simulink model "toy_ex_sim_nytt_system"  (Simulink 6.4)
settings: Solver=ode4  StartTime=0.0  StopTime=200  RelTol=1e-5
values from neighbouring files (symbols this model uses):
  alpha = -0.9    [bounds.m]    (also in real_ex_linkomb_W_and_DP.m = 1; real_ex_linkomb_W_and_RHOT.m = -0.2; real_ex_without_noise_z_30.m = -6:0.01:4; toy_ex_nytt_system.m)
  den_G1 = [-1 1]    [bounds.m]    (also in toy_ex_nytt_system.m; toy_ex_nytt_system_without_noise.m; toy_ex_nytt_system_with_disturbance.m; toy_ex_nytt_system_with_measure_noise.m)
  den_G2 = [-1 1]    [bounds.m]    (also in toy_ex_nytt_system.m; toy_ex_nytt_system_without_noise.m; toy_ex_nytt_system_with_disturbance.m; toy_ex_nytt_system_with_measure_noise.m)
  K = 2    [toy_ex_OLD.m]
  K_indre = 10    [real_ex_linkomb_W_and_DP.m]    (also in real_ex_linkomb_W_and_RHOT.m = 5; toy_ex_nytt_system.m = 50; toy_ex_nytt_system_without_noise.m = 20; toy_ex_nytt_system_with_disturbance.m = 50)
  num_G1 = 5*[-1.5 1]    [bounds.m]    (also in toy_ex_nytt_system.m; toy_ex_nytt_system_without_noise.m; toy_ex_nytt_system_with_disturbance.m; toy_ex_nytt_system_with_measure_noise.m)
  num_G2 = 5*[-0.5 1]    [bounds.m]    (also in toy_ex_nytt_system.m; toy_ex_nytt_system_without_noise.m; toy_ex_nytt_system_with_disturbance.m; toy_ex_nytt_system_with_measure_noise.m)
undefined symbols (not defined in the file or in its folder): Ti_indre

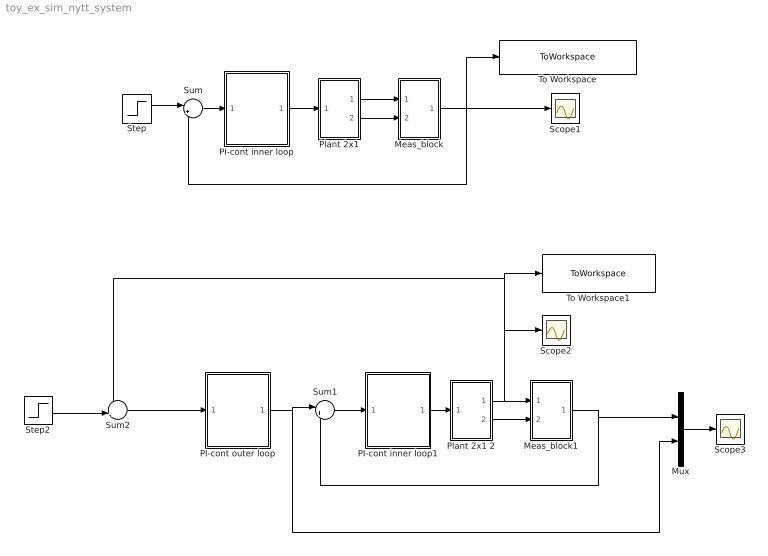
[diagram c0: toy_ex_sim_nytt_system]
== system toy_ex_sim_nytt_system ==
  Meas_block : Subsystem
  Meas_block1 : Subsystem
  Mux : Mux  Inputs=2
  PI-cont inner loop : Subsystem
  PI-cont inner loop1 : Subsystem
  PI-cont outer loop : Subsystem
  Plant 2x1 : Subsystem
  Plant 2x1 2 : Subsystem
  Scope1 : Scope
  Scope2 : Scope
  Scope3 : Scope
  Step : Step  SampleTime=0
  Step2 : Step  Time=20  SampleTime=0
  Sum : Sum  Inputs=|+-
  Sum1 : Sum  Inputs=|+-
  Sum2 : Sum  Inputs=-+|
  To Workspace : ToWorkspace  VariableName=meas_linkomb  SampleTime=-1  SaveFormat=Structure With Time
  To Workspace1 : ToWorkspace  VariableName=meas_linkomb1  SampleTime=-1  SaveFormat=Structure With Time
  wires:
  Plant 2x1/2(y2) -> Meas_block/2(In2)
  Plant 2x1/1("y1 ") -> Meas_block/1(In1)
  Meas_block/1(Out1) -> Sum/2, Scope1/1, To Workspace/1
  Step/1 -> Sum/1
  Sum/1 -> PI-cont inner loop/1(In1)
  PI-cont inner loop/1(Out1) -> Plant 2x1/1(In1)
  Plant 2x1 2/2(y2) -> Meas_block1/2(In2)
  Plant 2x1 2/1("y1 ") -> Meas_block1/1(In1), Sum2/1, To Workspace1/1, Scope2/1
  Meas_block1/1(Out1) -> Sum1/2, Mux/1
  Sum1/1 -> PI-cont inner loop1/1(In1)
  PI-cont inner loop1/1(Out1) -> Plant 2x1 2/1(In1)
  PI-cont outer loop/1(Out1) -> Sum1/1, Mux/2
  Step2/1 -> Sum2/2
  Sum2/1 -> PI-cont outer loop/1(In1)
  Mux/1 -> Scope3/1

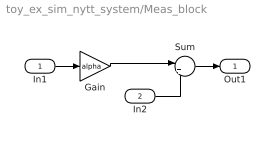
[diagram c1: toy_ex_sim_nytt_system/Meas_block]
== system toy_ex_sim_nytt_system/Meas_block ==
  In1 : Inport
  In2 : Inport  Port=2
  Gain : Gain  Gain=alpha
  Sum : Sum  Inputs=|++
  Out1 : Outport
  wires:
  Gain/1 -> Sum/1
  In1/1 -> Gain/1
  Sum/1 -> Out1/1
  In2/1 -> Sum/2

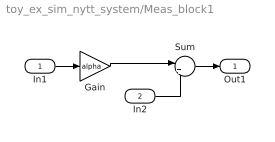
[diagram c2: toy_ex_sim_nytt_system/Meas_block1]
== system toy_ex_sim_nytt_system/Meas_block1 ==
  In1 : Inport
  In2 : Inport  Port=2
  Gain : Gain  Gain=alpha
  Sum : Sum  Inputs=|++
  Out1 : Outport
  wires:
  In2/1 -> Sum/2
  Sum/1 -> Out1/1
  In1/1 -> Gain/1
  Gain/1 -> Sum/1

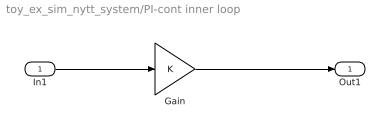
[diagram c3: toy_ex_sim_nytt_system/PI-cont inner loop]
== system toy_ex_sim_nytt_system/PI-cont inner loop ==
  In1 : Inport
  Gain : Gain  Gain=K
  Out1 : Outport
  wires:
  Gain/1 -> Out1/1
  In1/1 -> Gain/1

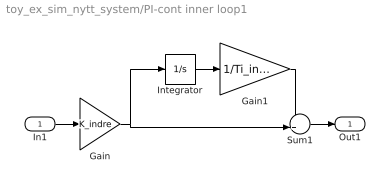
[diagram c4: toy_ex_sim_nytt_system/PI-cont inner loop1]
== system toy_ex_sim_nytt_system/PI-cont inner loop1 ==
  In1 : Inport
  Gain : Gain  Gain=K_indre
  Gain1 : Gain  Gain=1/Ti_indre
  Integrator : Integrator
  Sum1 : Sum  Inputs=++|
  Out1 : Outport
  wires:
  Sum1/1 -> Out1/1
  In1/1 -> Gain/1
  Gain1/1 -> Sum1/1
  Integrator/1 -> Gain1/1
  Gain/1 -> Sum1/2, Integrator/1

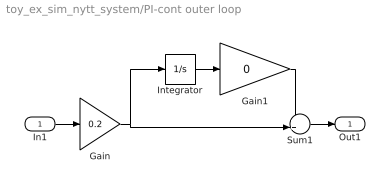
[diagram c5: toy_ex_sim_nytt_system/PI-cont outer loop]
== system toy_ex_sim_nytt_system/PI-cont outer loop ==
  In1 : Inport
  Gain : Gain  Gain=0.2
  Gain1 : Gain  Gain=0
  Integrator : Integrator
  Sum1 : Sum  Inputs=++|
  Out1 : Outport
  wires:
  Gain/1 -> Integrator/1, Sum1/2
  Integrator/1 -> Gain1/1
  Gain1/1 -> Sum1/1
  In1/1 -> Gain/1
  Sum1/1 -> Out1/1

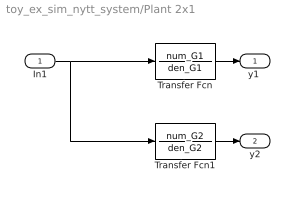
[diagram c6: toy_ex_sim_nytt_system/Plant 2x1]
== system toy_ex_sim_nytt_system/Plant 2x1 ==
  In1 : Inport
  Transfer Fcn : TransferFcn  Numerator=num_G1  Denominator=den_G1
  Transfer Fcn1 : TransferFcn  Numerator=num_G2  Denominator=den_G2
  "y1 " : Outport
  y2 : Outport  Port=2
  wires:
  In1/1 -> Transfer Fcn1/1, Transfer Fcn/1
  Transfer Fcn/1 -> "y1 "/1
  Transfer Fcn1/1 -> y2/1

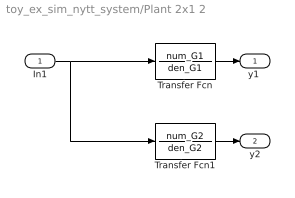
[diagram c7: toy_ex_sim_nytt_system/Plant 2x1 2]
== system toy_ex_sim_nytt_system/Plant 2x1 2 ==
  In1 : Inport
  Transfer Fcn : TransferFcn  Numerator=num_G1  Denominator=den_G1
  Transfer Fcn1 : TransferFcn  Numerator=num_G2  Denominator=den_G2
  "y1 " : Outport
  y2 : Outport  Port=2
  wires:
  Transfer Fcn1/1 -> y2/1
  Transfer Fcn/1 -> "y1 "/1
  In1/1 -> Transfer Fcn/1, Transfer Fcn1/1
